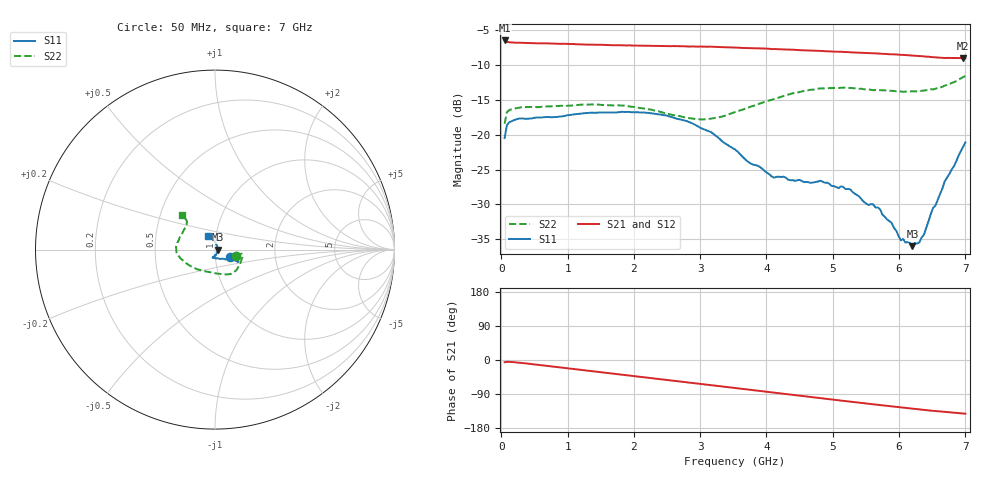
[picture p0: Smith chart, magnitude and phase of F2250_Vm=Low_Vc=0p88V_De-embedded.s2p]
! Integrated Device Technology
! Corporate Headquarters
! 6024 Silver Creek Valley Road
! San Jose, CA 95138  USA
! Phone:  1-408-284-8200
! Toll Free:  1-800-223-1366
! Webpage:  http://www.idt.com/
! Timing and RF Division
! 515 Groton Road, Suite 102
! Westford, MA 01886-6024
! Device:  F2250
! Description: Voltage Variable RF Attenuator
! Frequency:  50.0 -  6000.00 MHz
! Package:  3x3 mm Thin QFN Plastic Package: 16 pin
! Ports:  2 RF, 3 DC
!  Pin  1  = GND
!  Pin  2  = NC
!  Pin  3  = RF1  = Port 1
!  Pin  4  = NC
!  Pin  5  = GND
!  Pin  6  = GND
!  Pin  7  = GND
!  Pin  8  = GND
!  Pin  9  = NC
!  Pin 10  = RF2  = Port 2
!  Pin 11  = NC
!  Pin 12  = GND
!  Pin 13  = GND
!  Pin 14  = VCNTRL
!  Pin 15  = VDD
!  Pin 16  = VMODE
! Vcntrl:  0.880 Volts
! Vmode:  +0.000 Volts
! Vdd:  +3.30  Volts
! Current:  1.173 mA
! Data:  The device was measured on a the F2250 evaluation board which has
!  individual transmission lines to the RF pins.  Data was collected
!  using a calibrated network analyzer.  The evaluation board was
!  de-embedded using a TRL calibration technique.
!  The reference plane is the edge of the package pin.
! Misc:  SN 10
!  Action Tracker AT0258
! Date Measured:  2014-11-26
! Date:  2015-10-15  MJV
! Note:
!  Integrated Device Technology supplies this data as a sample of measured
!  data at the package pin for this product.  Your particular data for this
!  product may vary.
!  Data was taken at 25 degrees C.
!  Integrated Device Technology reserves the right to change this data at anytime.
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# GHz S dB R 50
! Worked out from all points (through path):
!   201 points, 50 MHz to 7 GHz, reference 50 ohm
!   highest |S21| = -6.47 dB at 50 MHz (marker M1); lowest = -9.0 dB at 6.965 GHz (marker M2)
!   group delay of S21, straight-line fit = 56.7 ps
!   lowest |S11| = -36.0 dB at 6.201 GHz (marker M3), VSWR 1.03, Z = 51.6 - j0.0227 ohm
!   |S11| at or under -10 dB: start of sweep to end of sweep
!   |S22| runs from -18.4 to -11.5 dB; largest |S21 - S12| = 0.0016
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0.05  -20.47 -24.4  -6.47 -5.9  -6.48 -5.9  -18.41 -17.9
0.08475  -18.62 -12.2  -6.67 -4.8  -6.67 -4.8  -16.76 -10.2
0.22375  -17.79 -8.4  -6.80 -6.2  -6.78 -6.2  -16.19 -10.8
1.2315  -16.93 -24.4  -7.04 -26.6  -7.03 -26.6  -15.67 -42.4
2.37825  -17.06 -27.7  -7.26 -49.8  -7.26 -49.8  -16.65 -70.1
3.0385  -19.15 -31.6  -7.36 -63.6  -7.36 -63.6  -17.81 -101.3
3.525  -22.11 -43.8  -7.49 -73.9  -7.47 -74.0  -16.75 -130.1
4.11575  -26.16 -77.7  -7.70 -86.4  -7.70 -86.4  -14.87 -156.8
4.7065  -26.84 -105.1  -7.93 -98.6  -7.93 -98.6  -13.53 -173.3
4.81075  -26.58 -106.0  -7.96 -100.7  -7.97 -100.7  -13.36 -175.4
5.2625  -27.82 -99.8  -8.18 -109.9  -8.18 -109.9  -13.28 174.1
5.50575  -29.89 -89.4  -8.26 -114.8  -8.26 -114.8  -13.51 168.2
5.6795  -30.43 -80.3  -8.34 -118.3  -8.34 -118.3  -13.60 163.6
5.85325  -32.38 -64.6  -8.45 -121.7  -8.44 -121.7  -13.70 159.1
6.027  -35.13 -44.2  -8.54 -125.1  -8.52 -125.2  -13.79 153.7
6.20075  -35.98 -0.8  -8.64 -128.6  -8.64 -128.6  -13.76 148.0
6.305  -35.44 33.7  -8.72 -130.5  -8.71 -130.6  -13.71 144.5
6.3745  -34.34 48.9  -8.76 -131.9  -8.76 -131.9  -13.66 142.2
6.5135  -30.47 74.2  -8.87 -134.1  -8.88 -134.2  -13.49 138.3
6.68725  -26.70 91.8  -8.99 -136.8  -8.99 -136.9  -12.95 134.5
6.96525  -21.72 115.4  -9.04 -141.2  -9.03 -141.2  -11.74 133.7
7  -21.12 116.9  -9.03 -141.7  -9.03 -141.8  -11.55 133.2
